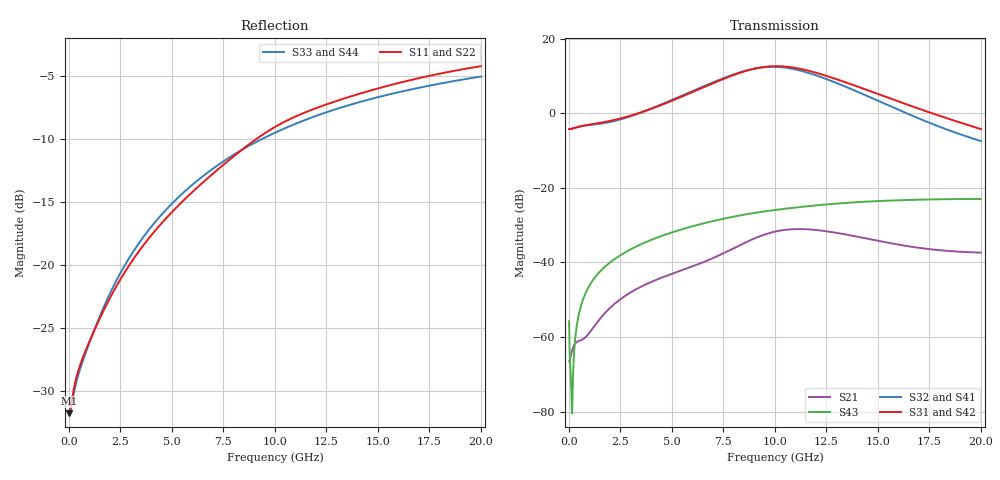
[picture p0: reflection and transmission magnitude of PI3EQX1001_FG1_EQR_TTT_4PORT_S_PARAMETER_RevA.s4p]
! NPort=4 DATA=2000 NOISE=0 GROUPDELAY=0 COMPLEX_DATAFORMAT=POLAR
! NumOfBlock=1 NumOfParam=0
! .MODEL Smodel S TSTONEFILE=PI3EQX1001_FG1_EQR_TTT_4PORT_S_PARAMETER_RevA.s4p TYPE=S
!  -- The above .MODEL line can be used for the S element in the netlist.
! The s parameter is extracted from the linear redriver, it is not bi-directional; only s(4,1)s(4,2) and s(3,1)s(3,2)
! should be the insertion loss
!Port definition:
!Port1 = input+
!Port2 = input¨C
!Port3 = output+
!Port4 = output-
# Hz S MA R  50
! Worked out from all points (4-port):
!   2000 points, 10 MHz to 20 GHz, reference 50 ohm
!   strongest paths, dB at 10 MHz, 5.01 GHz, 10.01 GHz, 15.01 GHz, 20 GHz:
!     S31: -4.3, 3.3, 12.6, 5.1, -4.3
!     S42: -4.3, 3.3, 12.6, 5.1, -4.3
!     S32: -4.3, 3.6, 12.4, 3.3, -7.5
!     S41: -4.3, 3.5, 12.4, 3.3, -7.5
!     S43: -55.8, -32.0, -26.0, -23.6, -23.0
!     S21: -66.5, -43.1, -31.8, -34.2, -37.4
!   lowest |S11| = -31.7 dB at 10 MHz (marker M1), VSWR 1.05, Z = 47.5 - j0.063 ohm
!   |S11| at or under -10 dB: start of sweep to 9.111 GHz
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1e7  0.02591 -178.5  0.0004939 2.7  3.669e-05 -0.2  4.787e-05 -0.1
     0.0004742 2.9  0.02597 -178.7  4.577e-05 -0.2  5.994e-05 -0.1
     0.6119 -0.4  0.6119 179.6  0.02616 178.4  0.001614 -59.2
     0.6116 179.6  0.6116 -0.4  0.001627 -58.9  0.02612 178.4
7.03e9  0.2317 -106.1  0.01081 78.2  2.194e-05 -30.8  3.228e-05 -29.6
        0.01151 76.6  0.2298 -106.1  2.905e-05 -25.8  4.003e-05 -25.0
        2.538 -58.6  2.608 126.3  0.2422 -112.0  0.03597 55.4
        2.6 126.4  2.538 -58.5  0.03592 55.6  0.2421 -112.0
9.03e9  0.3128 -107.7  0.02006 63.7  1.989e-05 -27.6  3.308e-05 -33.4
        0.02104 62.0  0.3106 -107.7  3.033e-05 -26.2  3.777e-05 -23.7
        3.954 -114.6  3.957 70.1  0.3055 -114.7  0.04606 42.8
        3.942 70.3  3.956 -114.5  0.04608 42.8  0.3053 -114.7
1.07e10  0.3775 -112.0  0.02647 34.4  2.207e-05 -21.8  3.394e-05 -44.4
         0.0276 32.9  0.3748 -112.1  3.178e-05 -35.9  4.029e-05 -21.7
         4.151 -172.6  3.993 12.4  0.3543 -117.3  0.05309 32.2
         3.978 12.6  4.153 -172.6  0.05309 32.2  0.3539 -117.3
1.304e10  0.4479 -117.5  0.02369 -0.1  2.911e-05 -36.9  2.965e-05 -64.8
          0.02473 -1.4  0.4442 -117.6  2.783e-05 -54.1  4.694e-05 -33.2
          2.822 117.6  2.504 -55.7  0.4165 -121.1  0.06152 17.7
          2.493 -55.4  2.821 117.6  0.06144 17.7  0.4164 -121.1
1.562e10  0.5164 -122.4  0.01717 -16.4  2.869e-05 -69.6  2.149e-05 -93.0
          0.01805 -17.9  0.5121 -122.4  1.933e-05 -77.7  4.369e-05 -56.0
          1.565 61.0  1.233 -107.2  0.4756 -125.1  0.06739 1.8
          1.228 -106.7  1.565 61.1  0.06733 1.8  0.4753 -125.1
2e10  0.6133 -130.1  0.01296 -15.5  1.505e-05 -148.7  1.243e-05 146.0
      0.01349 -18.3  0.6078 -130.2  7.623e-06 126.6  1.814e-05 -94.0
      0.611 -8.2  0.4226 -156.1  0.5579 -131.2  0.07075 -23.2
      0.423 -155.2  0.6105 -8.2  0.07072 -23.2  0.5578 -131.1
